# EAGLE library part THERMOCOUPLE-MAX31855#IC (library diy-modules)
Thermocouple Analog-to-Digital Converter based on MAX31855 chip Symbol with thermocouple connector pins MAX31855 datasheet available here: https://www.maximintegrated.com/en/products/analog/sensors-and-sensor-interface/MAX31855.html Click here to find device on ebay.com
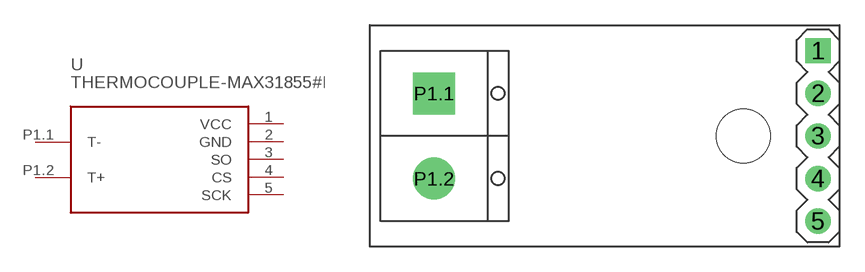
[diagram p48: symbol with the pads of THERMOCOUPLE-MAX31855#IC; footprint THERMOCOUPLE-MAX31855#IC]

Designator prefix -

## THERMOCOUPLE-MAX31855#IC  [THERMOCOUPLE-MAX31855#IC]
1  VCC  pwr
2  GND  out
3  SO
4  CS
5  SCK
P1.1  T-
P1.2  T+

## Footprint THERMOCOUPLE-MAX31855#IC (pad centres in mm)
Thermocouple Analog-to-Digital Converter based on MAX31855 chip Footprint with thermocouple connector pins
drill 1 square: 1 12.7,5.08
drill 1: 2 12.7,2.54; 3 12.7,0; 4 12.7,-2.54; 5 12.7,-5.08
drill 1.2 pad 2.5 square: P1.1 -10.16,2.54
drill 1.2 pad 2.5: P1.2 -10.16,-2.54
hole 3.2 at 8.255,0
